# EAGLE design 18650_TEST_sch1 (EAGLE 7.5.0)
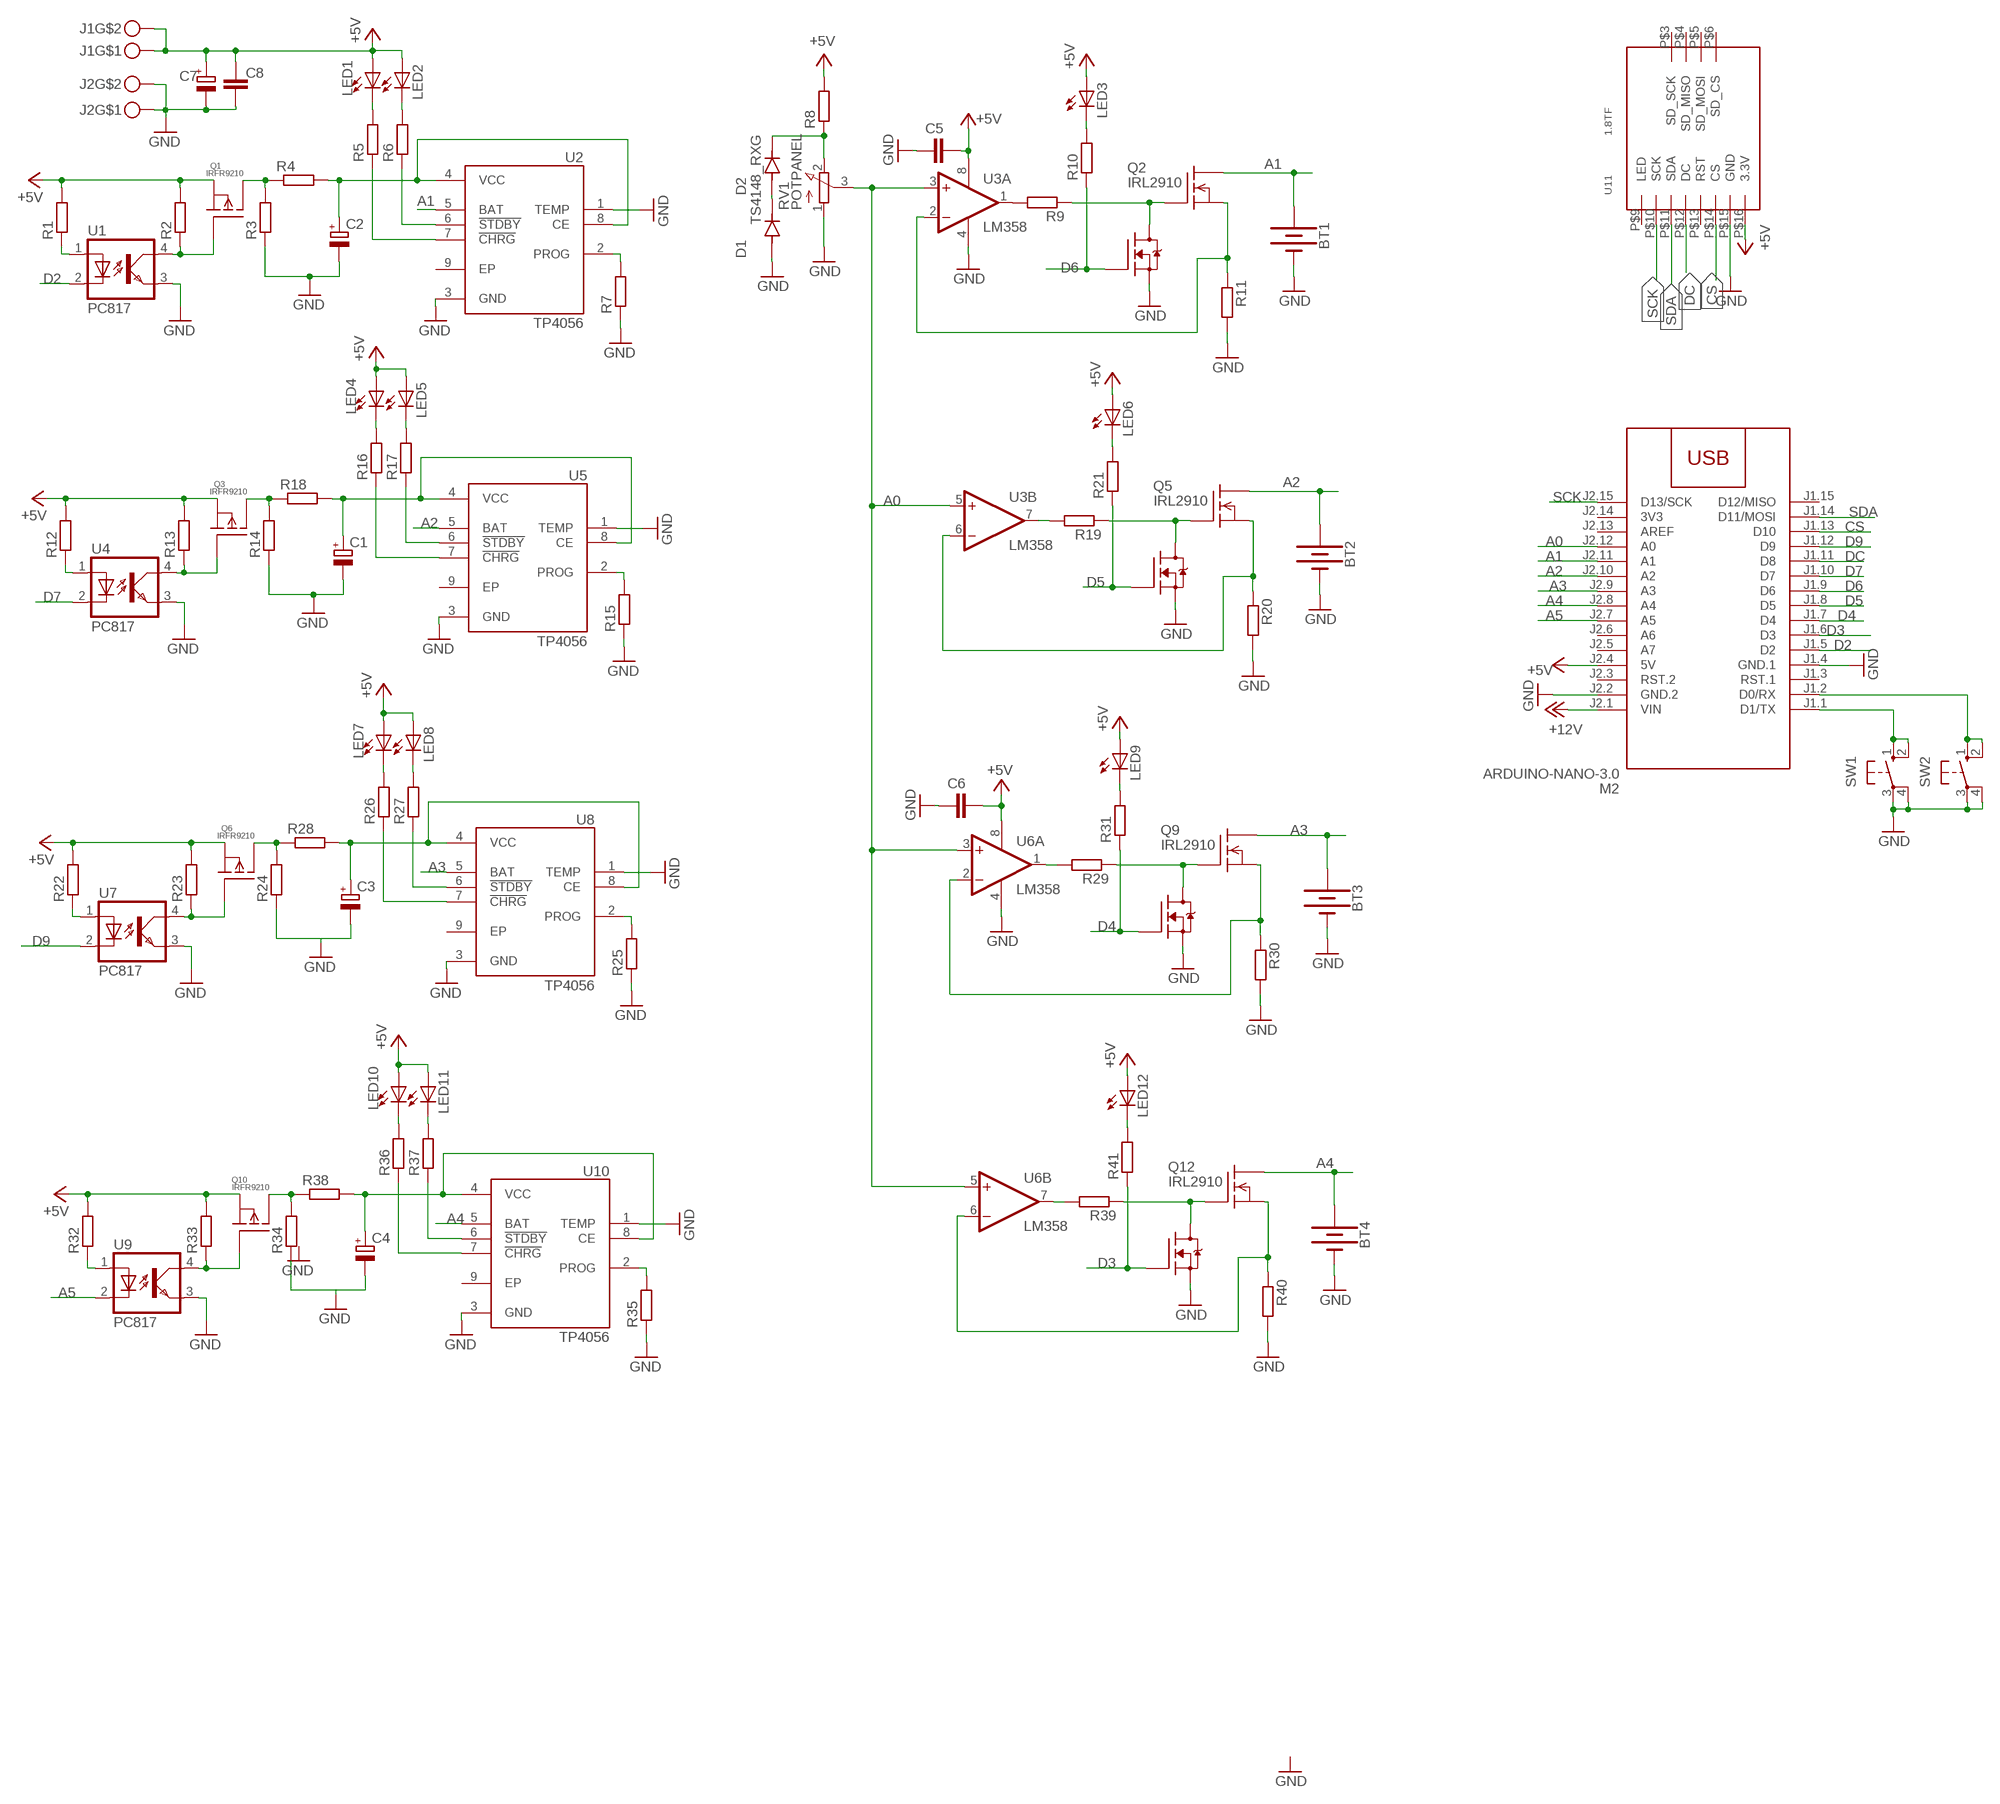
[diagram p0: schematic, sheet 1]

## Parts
BT1  BATTERY-18650  [BATTERY_18650-HOLDER]
BT2  BATTERY-18650  [BATTERY_18650-HOLDER]
BT3  BATTERY-18650  [BATTERY_18650-HOLDER]
BT4  BATTERY-18650  [BATTERY_18650-HOLDER]
C1  CPOL-EUSMCB  [SMC_B]
C2  CPOL-EUSMCB  [SMC_B]
C3  CPOL-EUSMCB  [SMC_B]
C4  CPOL-EUSMCB  [SMC_B]
C5  C-EUC1206  [C1206]
C6  C-EUC1206  [C1206]
C7  CPOL-EUSMCB  [SMC_B]
C8  C-EUC1206  [C1206]
D1  TS4148_RXG  [DIO_TS4148_RXG]
D2  TS4148_RXG  [DIO_TS4148_RXG]
J1  MKDSN1,5-2-5,08  [MKDSN1,5-2-5,08]
J2  MKDSN1,5-2-5,08  [MKDSN1,5-2-5,08]
LED1  LED5MM  [LED5MM]
LED2  LED5MM  [LED5MM]
LED3  LED5MM  [LED5MM]
LED4  LED5MM  [LED5MM]
LED5  LED5MM  [LED5MM]
LED6  LED5MM  [LED5MM]
LED7  LED5MM  [LED5MM]
LED8  LED5MM  [LED5MM]
LED9  LED5MM  [LED5MM]
LED10  LED5MM  [LED5MM]
LED11  LED5MM  [LED5MM]
LED12  LED5MM  [LED5MM]
M2  ARDUINO-NANO-3.0  [ARDUINO-NANO-3.0]
Q1  IRFR9210  [D2PACK]
Q2  IRL2910  SUP75N06-08  [TO220]
Q3  IRFR9210  [D2PACK]
Q4  ZVN3310F  [SOT23]
Q5  IRL2910  SUP75N06-08  [TO220]
Q6  IRFR9210  [D2PACK]
Q7  ZVN3310F  [SOT23]
Q8  ZVN3310F  [SOT23]
Q9  IRL2910  SUP75N06-08  [TO220]
Q10  IRFR9210  [D2PACK]
Q11  ZVN3310F  [SOT23]
Q12  IRL2910  SUP75N06-08  [TO220]
R1  R-EU_R1206  [R1206]
R2  R-EU_R1206  [R1206]
R3  R-EU_R1206  [R1206]
R4  R-EU_R2512  [R2512]
R5  R-EU_R1206  [R1206]
R6  R-EU_R1206  [R1206]
R7  R-EU_R1206  [R1206]
R8  R-EU_R1206  [R1206]
R9  R-EU_R1206  [R1206]
R10  R-EU_R1206  [R1206]
R11  R-EU_R2512  [R2512]
R12  R-EU_R1206  [R1206]
R13  R-EU_R1206  [R1206]
R14  R-EU_R1206  [R1206]
R15  R-EU_R1206  [R1206]
R16  R-EU_R1206  [R1206]
R17  R-EU_R1206  [R1206]
R18  R-EU_R2512  [R2512]
R19  R-EU_R1206  [R1206]
R20  R-EU_R2512  [R2512]
R21  R-EU_R1206  [R1206]
R22  R-EU_R1206  [R1206]
R23  R-EU_R1206  [R1206]
R24  R-EU_R1206  [R1206]
R25  R-EU_R1206  [R1206]
R26  R-EU_R1206  [R1206]
R27  R-EU_R1206  [R1206]
R28  R-EU_R2512  [R2512]
R29  R-EU_R1206  [R1206]
R30  R-EU_R2512  [R2512]
R31  R-EU_R1206  [R1206]
R32  R-EU_R1206  [R1206]
R33  R-EU_R1206  [R1206]
R34  R-EU_R1206  [R1206]
R35  R-EU_R1206  [R1206]
R36  R-EU_R1206  [R1206]
R37  R-EU_R1206  [R1206]
R38  R-EU_R2512  [R2512]
R39  R-EU_R1206  [R1206]
R40  R-EU_R2512  [R2512]
R41  R-EU_R1206  [R1206]
RV1  POTPANEL  [POTPANELP231]
SW1  40-XX  [B3F-40XX]
SW2  40-XX  [B3F-40XX]
U1  PC817  [DIL04]
U2  TP4056  [SOP127P600X175-9N]
U3  LM358  OPA2134PA  [DIL08]
U4  PC817  [DIL04]
U5  TP4056  [SOP127P600X175-9N]
U6  LM358  OPA2134PA  [DIL08]
U7  PC817  [DIL04]
U8  TP4056  [SOP127P600X175-9N]
U9  PC817  [DIL04]
U10  TP4056  [SOP127P600X175-9N]
U11  1.8TF  [1.8TFT]

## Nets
+5V: C5.1 C6.1 C7.+ C8.1 J1.1 J1.2 LED1.A LED2.A LED3.A LED4.A LED5.A LED6.A LED7.A LED8.A LED9.A LED10.A LED11.A LED12.A M2.J2.4(5V) Q1.3(S) Q3.3(S) Q6.3(S) Q10.3(S) R1.2 R2.2 R8.2 R12.2 R13.2 R22.2 R23.2 R32.2 R33.2 U3.8(A:V+) U6.8(A:V+) U11.P$16(3.3V)
+12V: M2.J2.1(VIN)
A0: M2.J2.12(A0) RV1.3(S) U3.3(A:+IN) U3.5(B:+IN) U6.3(A:+IN) U6.5(B:+IN)
A1: BT1.PWR@1(+) M2.J2.11(A1) Q2.2(D) U2.5(BAT)
A2: BT2.PWR@1(+) M2.J2.10(A2) Q5.2(D) U5.5(BAT)
A3: BT3.PWR@1(+) M2.J2.9(A3) Q9.2(D) U8.5(BAT)
A4: BT4.PWR@1(+) M2.J2.8(A4) Q12.2(D) U10.5(BAT)
A5: M2.J2.7(A5) U9.2(C)
CS: M2.J1.13(D10) U11.P$14(CS)
D2: M2.J1.5(D2) U1.2(C)
D3: M2.J1.6(D3) Q11.2(G) R41.1
D4: M2.J1.7(D4) Q8.2(G) R31.1
D5: M2.J1.8(D5) Q4.2(G) R21.1
D6: M2.J1.9(D6) Q7.2(G) R10.1
D7: M2.J1.10(D7) U4.2(C)
D9: M2.J1.12(D9) U7.2(C)
DC: M2.J1.11(D8) U11.P$12(DC)
GND: BT1.GND@1(-) BT2.GND@1(-) BT3.GND@1(-) BT4.GND@1(-) C1.- C2.- C3.- C4.- C5.2 C6.2 C7.- C8.2 D1.A J2.1 J2.2 M2.J1.4(GND.1) M2.J2.2(GND.2) Q4.3(S) Q7.3(S) Q8.3(S) Q11.3(S) R3.1 R7.1 R11.2 R14.1 R15.1 R20.2 R24.1 R25.1 R30.2 R34.1 R35.1 R40.2 RV1.1(A) SW1.3(P) SW1.4(P1) SW2.3(P) SW2.4(P1) U1.3(EMIT) U2.1(TEMP) U2.3(GND) U3.4(A:V-) U4.3(EMIT) U5.1(TEMP) U5.3(GND) U6.4(A:V-) U7.3(EMIT) U8.1(TEMP) U8.3(GND) U9.3(EMIT) U10.1(TEMP) U10.3(GND) U11.P$15(GND)
N$1: R7.2 U2.2(PROG)
N$2: LED1.K(C) R5.2
N$3: LED2.K(C) R6.2
N$4: R5.1 U2.7(!CHRG)
N$5: R6.1 U2.6(!STDBY)
N$6: Q1.2(D) R3.2 R4.1
N$7: M2.J1.1(D1/TX) SW1.1(S) SW1.2(S1)
N$8: M2.J1.2(D0/RX) SW2.1(S) SW2.2(S1)
N$9: R1.1 U1.1(A)
N$11: R12.1 U4.1(A)
N$12: Q1.1(G) R2.1 U1.4(COL)
N$13: C2.+ R4.2 U2.4(VCC) U2.8(CE)
N$14: Q3.1(G) R13.1 U4.4(COL)
N$15: C1.+ R18.2 U5.4(VCC) U5.8(CE)
N$16: R15.2 U5.2(PROG)
N$17: LED4.K(C) R16.2
N$18: LED5.K(C) R17.2
N$19: R16.1 U5.7(!CHRG)
N$20: R17.1 U5.6(!STDBY)
N$21: Q3.2(D) R14.2 R18.1
N$22: R19.2 U3.7(B:OUT)
N$23: Q4.1(D) Q5.1(G) R19.1
N$24: Q5.3(S) R20.1 U3.6(B:-IN)
N$25: LED6.K(C) R21.2
N$28: R22.1 U7.1(A)
N$29: Q6.1(G) R23.1 U7.4(COL)
N$30: C3.+ R28.2 U8.4(VCC) U8.8(CE)
N$31: R25.2 U8.2(PROG)
N$32: LED7.K(C) R26.2
N$33: LED8.K(C) R27.2
N$34: R26.1 U8.7(!CHRG)
N$35: R27.1 U8.6(!STDBY)
N$36: Q6.2(D) R24.2 R28.1
N$37: Q8.1(D) Q9.1(G) R29.1
N$38: Q9.3(S) R30.1 U6.2(A:-IN)
N$39: LED9.K(C) R31.2
N$40: R29.2 U6.1(A:OUT)
N$42: R32.1 U9.1(A)
N$43: Q10.1(G) R33.1 U9.4(COL)
N$44: C4.+ R38.2 U10.4(VCC) U10.8(CE)
N$45: R35.2 U10.2(PROG)
N$46: LED10.K(C) R36.2
N$47: LED11.K(C) R37.2
N$48: R36.1 U10.7(!CHRG)
N$49: R37.1 U10.6(!STDBY)
N$50: Q10.2(D) R34.2 R38.1
N$51: Q11.1(D) Q12.1(G) R39.1
N$52: Q12.3(S) R40.1 U6.6(B:-IN)
N$53: LED12.K(C) R41.2
N$55: R39.2 U6.7(B:OUT)
N$58: D2.C(K) R8.1 RV1.2(E)
N$59: D1.C(K) D2.A
N$60: R9.2 U3.1(A:OUT)
N$61: Q2.1(G) Q7.1(D) R9.1
N$62: Q2.3(S) R11.1 U3.2(A:-IN)
N$91: LED3.K(C) R10.2
SCK: M2.J2.15(D13/SCK) U11.P$10(SCK)
SDA: M2.J1.14(D11/MOSI) U11.P$11(SDA)
Unconnected: M2.J1.3(RST.1) M2.J1.15(D12/MISO) M2.J2.3(RST.2) M2.J2.5(A7) M2.J2.6(A6) M2.J2.13(AREF) U2.9(EP) U5.9(EP) U8.9(EP) U10.9(EP) U11.P$3(SD_SCK) U11.P$4(SD_MISO) U11.P$5(SD_MOSI) U11.P$6(SD_CS) U11.P$9(LED) U11.P$13(RST)

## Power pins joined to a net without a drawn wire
3V3: M2.J2.14(3V3)

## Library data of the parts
BT1-BT4 = SparkFun-Batteries:BATTERY: Battery - Single Cell; PROD_ID: BATT-12327; SF_SKU: PRT-13113
C1-C4 C7 = rcl:CPOL-EU: POLARIZED CAPACITOR, European symbol
C5 C6 C8 = rcl:C-EU: CAPACITOR, European symbol
D1 D2 = TS4148_RXG:TS4148_RXG: Check availability Check availability Check availability; AVAILABILITY: In Stock; CHECK_PRICES: https://www.snapeda.com/parts/TS4148%20RXG/Taiwan+Semiconductor/view-part/?ref=eda; DESCRIPTION: 1206 (Ceramics) 75V 0.15A Switching Diode & Array; MF: Taiwan Semiconductor; MP: TS4148 RXG; PACKAGE: 1206-2 Taiwan Semiconductor; PRICE: None; SNAPEDA_LINK: https://www.snapeda.com/parts/TS4148%20RXG/Taiwan+Semiconductor/view-part/?ref=snap
J1 J2 = con-phoenix-508:MKDSN1,5-2-5,08
LED1-LED12 = led:LED: LED
M2 = diy-modules:ARDUINO-NANO-3.0: Arduino Nano 3.0 and compatible devices More details available here: https://www.arduino.cc/en/Main/ArduinoBoardNano Click here to find device on ebay.com
Q1 Q3 Q6 Q10 = IRFR9210:IRFR9210: Check availability; AVAILABILITY: In Stock; CHECK_PRICES: https://www.snapeda.com/parts/IRFR9210/Vishay+Siliconix/view-part/?ref=eda; DESCRIPTION: P-Channel 200 V 1.9A (Tc) 2.5W (Ta), 25W (Tc) Surface Mount D-Pak; MF: Vishay; MP: IRFR9210; PACKAGE: TO-252-3 Infineon; PRICE: None; SNAPEDA_LINK: https://www.snapeda.com/parts/IRFR9210/Vishay+Siliconix/view-part/?ref=snap
Q2 Q5 Q9 Q12 = transistor-fet:SUP75N06-08: N-Channel Enhancement MOSFET 60V; 75A; 0,008Ohm
Q4 Q7 Q8 Q11 = transistor-fet:ZVN3310F
R1-R41 = rcl:R-EU_: RESISTOR, European symbol
RV1 = pot:POTPANEL
SW1 SW2 = switch-omron:40-XX: OMRON SWITCH; MF: OMRON COMPONENTS USA; MPN: B3F-4000; OC_FARNELL: 176434; OC_NEWARK: 36K3105
U1 U4 U7 U9 = optocoupler:PC817: SHARP OPTO COUPLER; MPN: PC817X4J000F; OC_FARNELL: 9707727; OC_NEWARK: 97K7059
U2 U5 U8 U10 = TP4056:TP4056: Check availability; AVAILABILITY: Not in stock; CHECK_PRICES: https://www.snapeda.com/parts/TP4056/NanJing+Top+Power+ASIC+Corp./view-part/?ref=eda; DESCRIPTION: Complete single cell Li-Ion battery with a constant current / constant voltage linear charger; MF: NanJing Top Power ASIC Corp.; MP: TP4056; PACKAGE: Package; PRICE: None; SNAPEDA_LINK: https://www.snapeda.com/parts/TP4056/NanJing+Top+Power+ASIC+Corp./view-part/?ref=snap
U3 U6 = linear:OPA2*: Dual Operational Amplifier Low Power, Single-Supply, Rail-To-Rail Operational Amplifier Source: http://focus.ti.com/lit/ds/symlink/opa2345.pdf http://focus.ti.com .. opa241.pdf http://focus.ti.com/lit/ds/symlink/opa2134.pdf
U11 = tft_1_8_1_44_oled_0_96:1.8TF

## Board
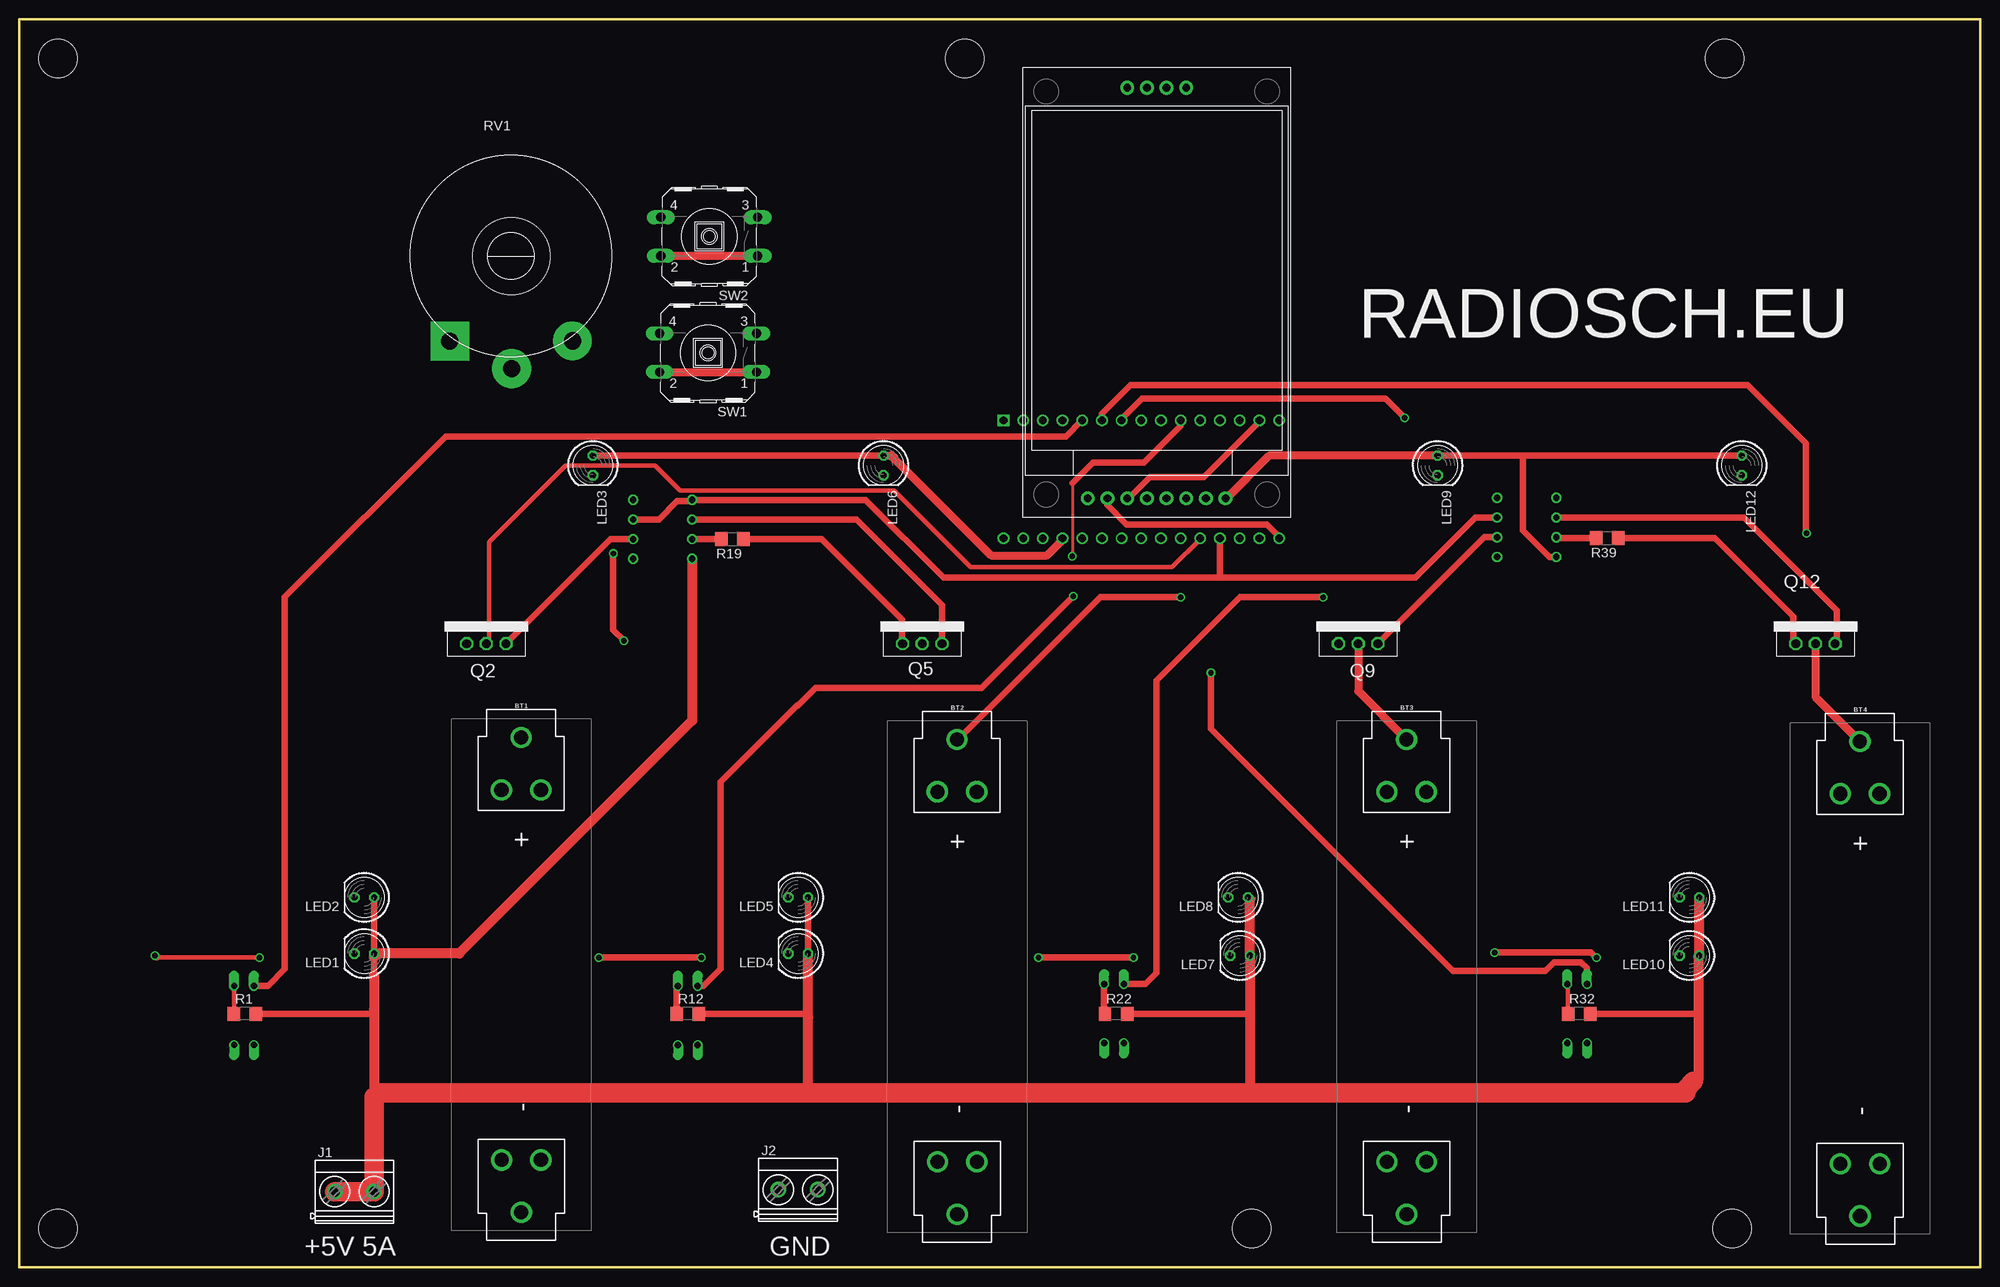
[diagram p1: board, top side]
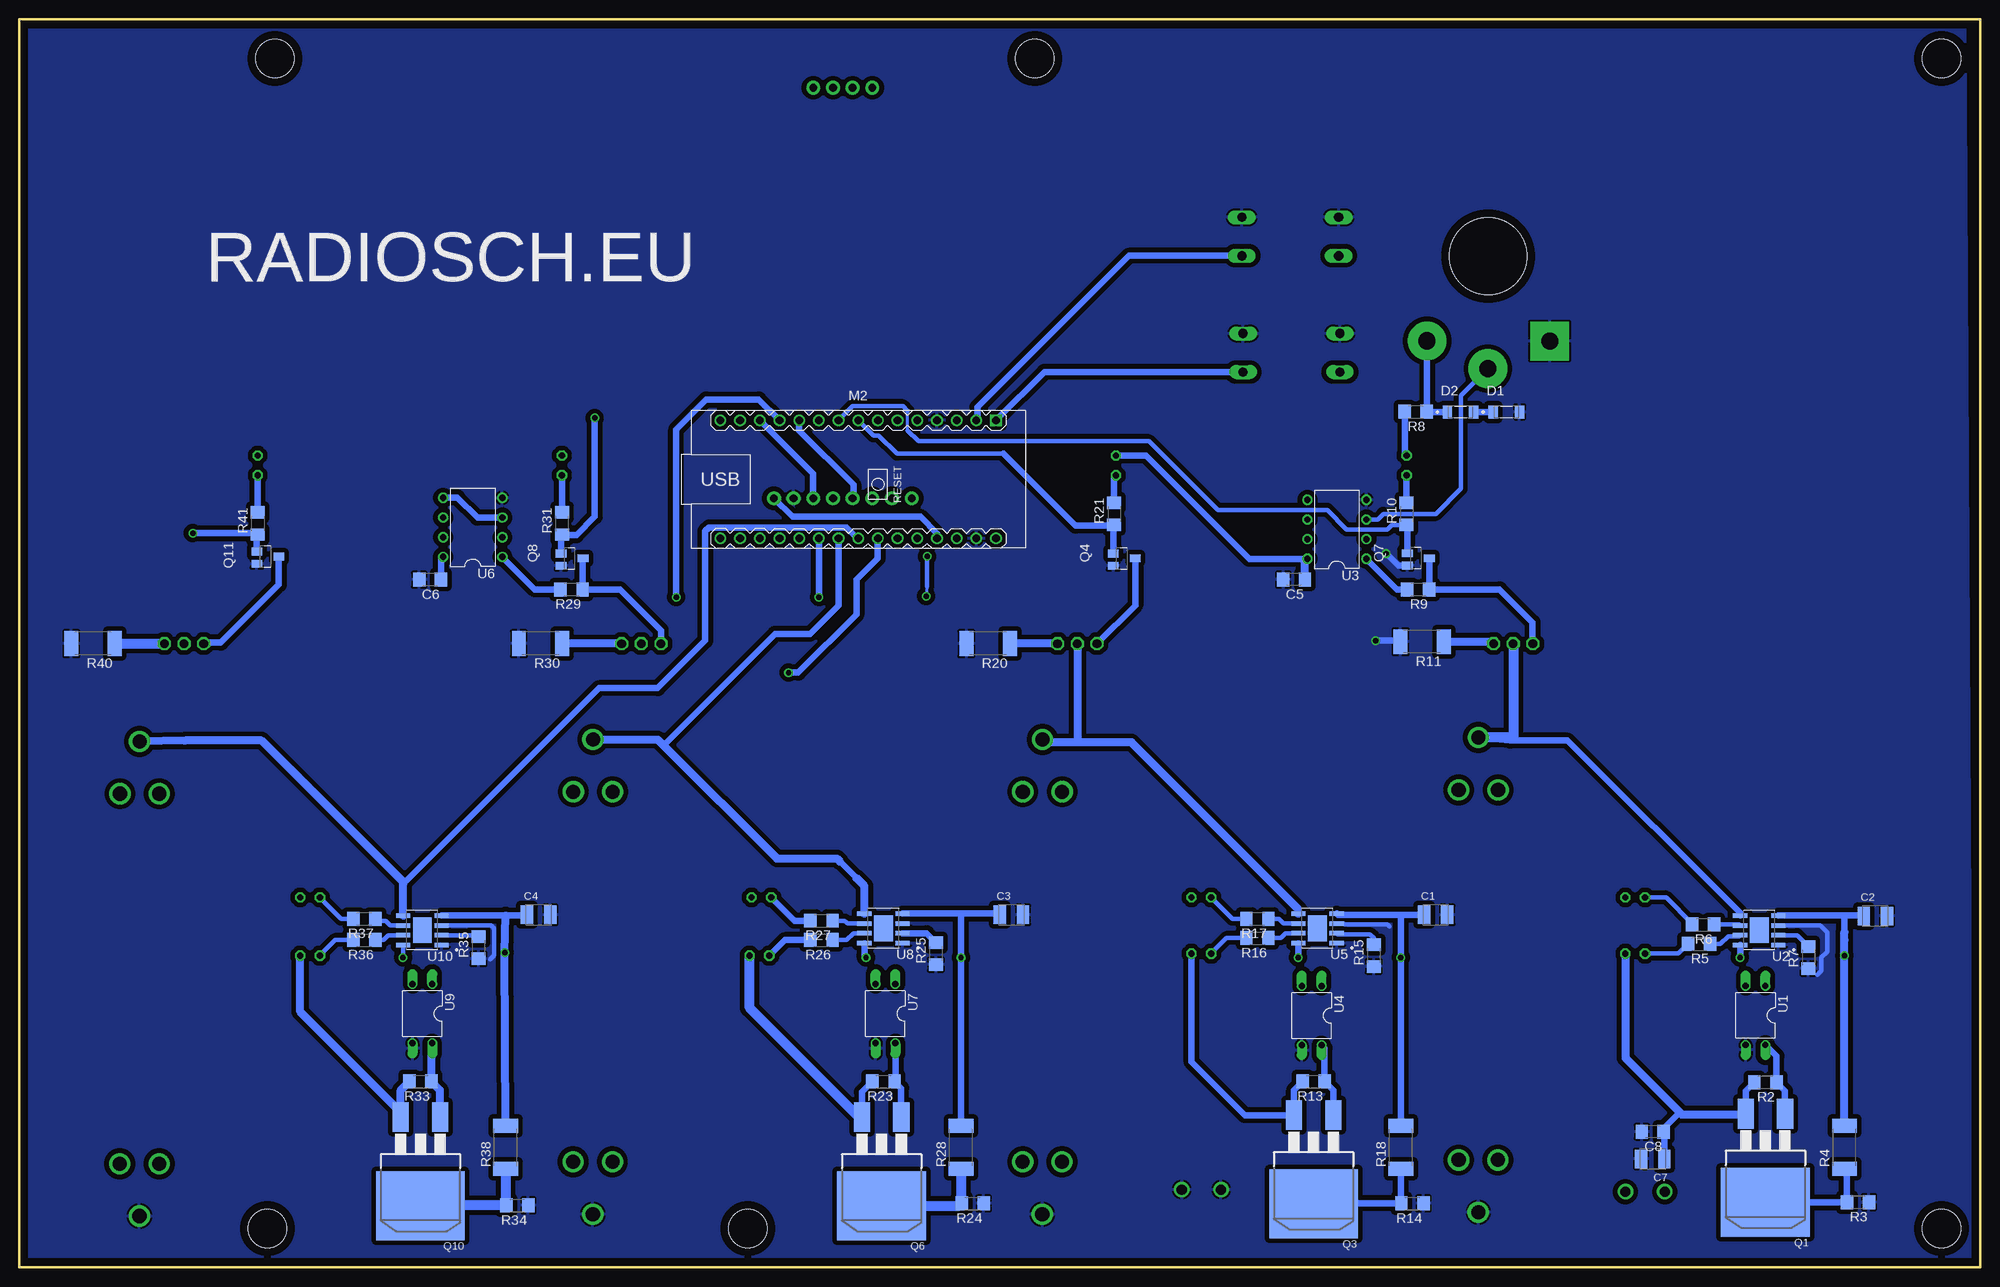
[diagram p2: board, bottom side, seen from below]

Size 253 x 161.06 mm. Coordinates in mm from the lower left corner, seen from the top.
Outline: 0,0 253,0 253,161.06 0,161.06 0,0
Copper layers (1*16): Top 0.035mm / dielectric 1.5mm / Bottom 0.035mm
Design rules "default": minimum track width 10mil, minimum drill 24mil, track to track 8mil, track to pad 8mil, pad to pad 8mil, via to via 8mil, smd to smd 8mil, copper to edge 40mil, drill to drill 8mil, minimum pad ring 10mil, minimum via ring 8mil, stop-mask expansion 4mil, vias tented up to drill 0mil, thermal gap 10mil
Holes 10 mm at 63.5,130.5
Holes 5 mm at 5,156 5,5 122,156 159,5 221,5 220,156

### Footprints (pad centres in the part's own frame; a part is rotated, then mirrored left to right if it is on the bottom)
BATTERY_18650-HOLDER = drill 1.829: GND@1 30.628,0.01; GND@2 23.88,2.55; GND@3 23.88,-2.53; PWR@1 -30.628,-0.01; PWR@2 -23.88,2.53; PWR@3 -23.88,-2.55
SMC_B = smd 1.6 x 2.4: + -1.5,0; - 1.5,0
C1206 = smd 1.6 x 1.8: 1 -1.4,0; 2 1.4,0
DIO_TS4148_RXG = smd 1.2 x 1.7: A 1.7,0; C -1.7,0
MKDSN1,5-2-5,08 = drill 1.3 pad 2: 1 -2.561,0.025; 2 2.519,0.025
LED5MM = drill 0.813 octagon: A -1.27,0; K 1.27,0
ARDUINO-NANO-3.0 = drill 1 square: J1.1 17.78,7.62 | drill 1: J1.2 15.24,7.62; J1.3 12.7,7.62; J1.4 10.16,7.62; J1.5 7.62,7.62; J1.6 5.08,7.62; J1.7 2.54,7.62; J1.8 0,7.62; J1.9 -2.54,7.62; J1.10 -5.08,7.62; J1.11 -7.62,7.62; J1.12 -10.16,7.62; J1.13 -12.7,7.62; J1.14 -15.24,7.62; J1.15 -17.78,7.62; J2.1 17.78,-7.62; J2.2 15.24,-7.62; J2.3 12.7,-7.62; J2.4 10.16,-7.62; J2.5 7.62,-7.62; J2.6 5.08,-7.62; J2.7 2.54,-7.62; J2.8 0,-7.62; J2.9 -2.54,-7.62; J2.10 -5.08,-7.62; J2.11 -7.62,-7.62; J2.12 -10.16,-7.62; J2.13 -12.7,-7.62; J2.14 -15.24,-7.62; J2.15 -17.78,-7.62
D2PACK = smd 2.083 x 3.81: 1 -2.54,-8.89; 3 2.54,-8.89 | smd 11.43 x 8.89: 2 0,2.54
TO220 = drill 1.118 octagon: 1 -2.54,0; 2 0,0; 3 2.54,0
SOT23 = smd 1 x 1.4: 1 0,1.735; 2 -0.632,-1.1; 3 0.95,-1.1
R1206 = smd 1.6 x 1.803: 1 -1.422,0; 2 1.422,0
R2512 = smd 1.8 x 3.2: 1 -2.8,0; 2 2.8,0
POTPANELP231 = drill 2.2 pad 5 square: 1 -7.85,-11 | drill 2.2 pad 5: 2 7.97,-10.96; 3 0.11,-14.54
B3F-40XX = drill 1.194 long: 1 -6.248,2.489; 2 6.248,2.489; 3 -6.248,-2.489; 4 6.248,-2.489
DIL04 = drill 0.813 offset: 1 -1.27,-3.81; 2 1.27,-3.81; 3 1.27,3.81; 4 -1.27,3.81
SOP127P600X175-9N = smd 1.97 x 0.6: 1 -2.475,1.905; 2 -2.475,0.635; 3 -2.475,-0.635; 4 -2.475,-1.905; 5 2.475,-1.905; 6 2.475,-0.635; 7 2.475,0.635; 8 2.475,1.905 | smd 2.413 x 3.302: 9 0,0
DIL08 = drill 0.813 pad 1.27: 1 -3.81,-3.81; 2 -1.27,-3.81; 3 1.27,-3.81; 4 3.81,-3.81; 5 3.81,3.81; 6 1.27,3.81; 7 -1.27,3.81; 8 -3.81,3.81
1.8TFT = drill 1 pad 1.778: P$3 55.5,21.05; P$4 55.5,18.52; P$5 55.5,15.98; P$6 55.5,13.44; P$9 2.5,26.14; P$10 2.5,23.6; P$11 2.5,21.06; P$12 2.5,18.52; P$13 2.5,15.98; P$14 2.5,13.44; P$15 2.5,10.9; P$16 2.5,8.36

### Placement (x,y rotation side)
BT1  64.75,37.75 270 top
BT2  121,37.5 270 top
BT3  179,37.5 270 top
BT4  237.5,37.25 270 top
C1  70.25,45.5 0 bottom
C2  13.51,45.35 0 bottom
C3  125,45.5 0 bottom
C4  186,45.5 0 bottom
C5  88.52,88.76 180 bottom
C6  200,88.75 180 bottom
C7  42.25,14 180 bottom
C8  42.25,17.5 180 bottom
D1  61.12,110.39 0 bottom
D2  67.05,110.39 0 bottom
J1  43.25,9.75 0 top
J2  100.5,10 0 top
LED1  44.5,40.5 180 top
LED2  44.5,47.75 180 top
LED3  74,103.5 270 top
LED4  100.5,40.5 180 top
LED5  100.5,47.75 180 top
LED6  111.5,103.5 270 top
LED7  157.5,40.25 180 top
LED8  157.25,47.75 180 top
LED9  183,103.5 270 top
LED10  215.5,40.25 180 top
LED11  215.5,47.75 180 top
LED12  222.25,103.5 270 top
M2  144.76,101.7 0 bottom
Q1  27.71,10.93 180 bottom
Q2  60.25,80.5 0 top
Q3  86,10.75 180 bottom
Q4  110.75,91.5 270 bottom
Q5  116.5,80.5 0 top
Q6  141.75,10.5 180 bottom
Q7  72.81,91.52 270 bottom
Q8  182,91.5 270 bottom
Q9  172.75,80.5 0 top
Q10  201.25,10.5 180 bottom
Q11  221.25,91.75 270 bottom
Q12  231.75,80.5 0 top
R1  29.11,32.73 0 top
R2  27.71,23.9 180 bottom
R3  15.76,8.43 180 bottom
R4  17.5,15.5 90 bottom
R5  36.25,41.75 180 bottom
R6  35.75,44.25 180 bottom
R7  22.16,40 90 bottom
R8  72.81,110.43 180 bottom
R9  72.5,87.5 180 bottom
R10  74,97.25 90 bottom
R11  72,80.75 180 bottom
R12  86.25,32.75 0 top
R13  86,24 180 bottom
R14  73.25,8.25 180 bottom
R15  78.25,40.25 90 bottom
R16  93.25,42.5 180 bottom
R17  93.25,45 180 bottom
R18  74.75,15.5 90 bottom
R19  92,94 180 top
R20  128,80.5 180 bottom
R21  111.75,97.25 90 bottom
R22  141.5,32.75 0 top
R23  141.5,24 180 bottom
R24  130,8.25 180 bottom
R25  134.75,40.5 90 bottom
R26  149.5,42.25 180 bottom
R27  149.5,44.75 180 bottom
R28  131.5,15.5 90 bottom
R29  181.75,87.5 180 bottom
R30  185.75,80.5 180 bottom
R31  183,96 90 bottom
R32  201.25,32.75 0 top
R33  201.25,24 180 bottom
R34  188.75,8 180 bottom
R35  193.75,41.25 90 bottom
R36  208.5,42.25 180 bottom
R37  208.5,45 180 bottom
R38  190.25,15.5 90 bottom
R39  204.88,94.12 180 top
R40  243.5,80.5 180 bottom
R41  222.25,96 90 bottom
RV1  63.4,130.53 0 top
SW1  88.86,118.03 180 top
SW2  89.02,133.03 180 top
U1  28.98,32.52 180 bottom
U2  28.5,43.5 180 bottom
U3  83,95.25 90 bottom
U4  86.25,32.5 180 bottom
U5  85.5,43.75 180 bottom
U6  194.5,95.5 90 bottom
U7  141.25,32.75 180 bottom
U8  141.5,43.75 180 bottom
U9  201,32.75 180 bottom
U10  201,43.5 180 bottom
U11  164,96.75 90 top

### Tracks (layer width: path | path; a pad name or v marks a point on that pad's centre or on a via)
+5V
  Top 0.813: 45.77,37.75 45.77,40 LED1.A LED2.A | LED5.A LED4.A 101.75,40.48 101.75,37 | R12.2 101.77,32.75 101.77,32.25 | R1.2 45.77,32.73 45.77,33.25 | R22.2 158.52,32.75 158.77,32.5 | R32.2 216.62,32.75 | LED3.A LED6.A | LED9.A 193.75,104.77 | 193.75,104.77 LED12.A | U6.8 197.44,91.69 194,95.12 194,104.52 193.75,104.77
  Top 1.016: LED6.A 112.48,104.77 125.38,91.88 132.62,91.88 134.6,93.85 M2.J2.4 | LED9.A 182.98,104.75 161.25,104.75 155.75,99.25 U11.P$16
  Top 1.27: 45.77,37.75 45.77,33.25 45.77,22 46.27,22.5 | 101.77,22.5 101.77,32.25 LED4.A | U3.8 86.81,70.56 56.75,40.5 46.27,40.5 45.77,40 | 159,22.5 158.77,22.73 158.77,32.5 LED7.A 158.77,47.5 LED8.A | LED11.A LED10.A 216.62,40.1 216.62,32.75 216.62,24.12 215,22.5 | J1.2
  Top 2.54: 46.27,22.5 101.77,22.5 159,22.5 214.5,22.5 215,23 | 45.77,22 J1.2 | J1.1 J1.2 | 215,23 216,24 | 215,22.5 215,23
  Bottom 0.813: Q1.3 30.25,22.78 R2.2 | R13.2 88.54,22.88 Q3.3 94.89,19.64 101.75,26.5 101.75,40.48 LED4.A | R23.2 144.29,22.63 Q6.3 | U3.8 94.3,91.44 107.62,104.77 LED6.A | C6.1 198.6,91.4 U6.8 | M2.J2.4 134.6,94.72 136.75,96.88 153.26,96.88 U11.P$16 | R8.2 74.24,105.01 LED3.A | C7.+ 40.75,17.4 C8.1 40.85,17.9 38.75,20
  Bottom 1.016: LED1.A 45.77,27.02 38.75,20 38.5,19.75 30.32,19.75 Q1.3 | C5.1 87.12,91.13 U3.8 | R33.2 203.79,22.88 Q10.3 203.79,20.04 216.75,33 216.75,40.23 LED10.A
  Bottom 1.27: Q6.3 144.66,19.39 158.77,33.5 LED7.A
A0
  Top 0.813: 79.17,96.5 U3.3 82.52,96.52 84.88,98.88 86.62,98.88 U3.5 109.19,99.06 119.25,89 155,89 | U6.3 190.67,96.75 187.88,96.75 180.12,89 155,89 | M2.J2.12 154.92,89.08 155,89
  Bottom 0.61: U3.3 77.73,96.52 77,97.25 70.25,97.25 67,100.5 67,112.5 RV1.3
  Bottom 0.813: U6.3 193.9,96.77 196.5,99.38 198.25,99.38 U6.5
A1
  Top 0.61: Q2.2 60.62,80.88 60.62,93.62 70.5,103.5 82,103.5 85.25,100.25 112.88,100.25 122.75,90.38 148.75,90.38 152.38,94 M2.J2.11
  Bottom 0.813: U2.5 30.98,45.73 53.25,68 60.62,68 BT1.PWR@1
  Bottom 1.27: Q2.2 60.25,68.37 BT1.PWR@1
A2  (via drill 0.7)
  Top 0.813: BT2.PWR@1 120.88,67.88 139.5,86.5 v149.84,86.5
  Bottom 0.813: v149.84,86.5 M2.J2.10
  Bottom 1.016: U5.5 87.97,46.23 109.5,67.75 116.25,67.75 | Q5.2 116.49,67.99 116.25,67.75 | 116.25,67.75 120.61,67.75 BT2.PWR@1
A3
  Top 1.016: Q9.2 172.75,74.37 BT3.PWR@1
  Bottom 0.813: 147.3,52.55 147.12,52.38 145,50.25 | M2.J2.9 147.3,85.45 151,81.75 155.5,81.75 169.88,67.38
  Bottom 1.016: U8.5 143.97,49.23 145,50.25 | BT3.PWR@1 170.63,68.13 169.88,67.38 155.25,52.75 147.5,52.75 147.12,52.38
A4
  Top 1.016: Q12.2 231.75,73.62 BT4.PWR@1
  Bottom 0.813: M2.J2.8 144.83,94.08 146.25,95.5 164,95.5 164.5,95 164.5,80.88 170.62,74.75 178.22,74.75 203.47,49.5
  Bottom 1.016: U10.5 203.47,49.5 203.47,49.73 221.75,68 231.61,68 BT4.PWR@1
A5  (via drill 0.7)
  Top 0.813: U9.2 202.25,36.58 202.25,38.62 201.5,39.38 198,39.38 196.88,38.25 185,38.25 153.75,69.5 v153.75,76.75
  Bottom 0.813: M2.J2.7 142.25,94.05 142.25,91.5 145,88.75 145,84.25 152.5,76.75 v153.75,76.75
CS
  Bottom 0.813: U11.P$14 150.56,102.42 M2.J1.13
D2
  Top 0.813: U1.2 32.08,36.33 34.25,38.5 34.25,86.5 55,107.25 135.07,107.25 M2.J1.5 137,109.46
D3  (via drill 0.7)
  Top 0.813: M2.J1.6 139.68,110.18 143.38,113.88 223,113.88 230.5,106.38 230.5,94.88 v230.62,94.75
  Bottom 0.813: Q11.2 222.35,94.48 R41.1 222.42,94.75 v230.62,94.75
D4  (via drill 0.7)
  Top 0.813: M2.J1.7 142.22,109.47 144.88,112.12 176.25,112.12 v178.75,109.62
  Bottom 0.813: Q8.2 183.1,94.48 R31.1 182.92,94.5 181.12,94.5 178.75,96.88 v178.75,109.62
D5
  Bottom 0.61: M2.J1.8 142.81,107.38 142.12,107.38 139.75,105 126,105
  Bottom 0.813: Q4.2 111.85,95.73 | 111.85,95.73 R21.1 | 111.85,95.73 116.73,95.73 126,105
D6
  Bottom 0.406: 138.38,108 138.38,110.5
  Bottom 0.61: R10.1 75.92,95.83 76.5,95.25 81.75,95.25 84.25,97.75 98.38,97.75 107.25,106.62 137,106.62 138.38,108 | 138.38,110.5 139,111.12 145.5,111.12 M2.J1.9
  Bottom 0.813: Q7.2 73.91,95.74 R10.1
D7  (via drill 0.7)
  Top 0.406: 135.88,101.25 v135.88,91.75
  Top 0.813: U4.2 88.31,36.31 90.5,38.5 90.5,62.62 100.38,72.5 100.5,72.5 102.75,74.75 124.12,74.75 v136,86.62 | M2.J1.10 149.84,108.59 145.12,103.88 138.5,103.88 135.88,101.25
  Bottom 0.406: 135.88,87.88 v136,86.62
  Bottom 0.61: v135.88,91.75 135.88,87.88
D9  (via drill 0.7)
  Top 0.813: U7.2 145.31,36.56 146.75,38 146.75,75.75 157.5,86.5 v168.25,86.5
  Bottom 0.813: v168.25,86.5 168.25,108.12 164.38,112 157.6,112 M2.J1.12
DC
  Bottom 0.813: M2.J1.11 152.38,108 145.38,101 145.38,99.36 U11.P$12
GND  (via drill 0.7)
  Top 0.813: v76.62,92.12 76.62,82.25 v78,80.88
  Bottom 0.61: U2.3 20.64,44.13 19.75,43.25 19.75,40.75 20.5,40 20.5,38.25 21,37.75 | U5.3 82.14,44.38 82,44.25 76.5,44.25 76.25,44 | U10.3 192.13,44.13 191.75,43.75 191.75,40.25 192.25,39.75
  Bottom 0.813: Q7.3 75.07,90.57 v76.62,92.12 | v78,80.88 74.92,80.88 R11.2
  pour Bottom (isolate 0.61): 2,174 292,173 291,-2 1,-1
N$1
  Bottom 0.61: U2.2 23.6,42.87 R7.2
N$2
  Bottom 0.61: LED1.K 38.92,40.5 R5.2
N$3
  Bottom 0.61: R6.2 37.17,44.42 40.5,47.75 LED2.K
N$4
  Bottom 0.61: R5.1 33.5,41.75 32.5,42.75 31.09,42.75 U2.7
N$5
  Bottom 0.61: R6.1 31.09,44.25 U2.6
N$6
  Bottom 0.813: Q1.2 17.22,8.39 R3.2 17.18,12.38 R4.1
N$7
  Top 1.016: SW1.2 SW1.1
  Bottom 0.813: SW1.1 120.75,115.55 M2.J1.1
N$8
  Top 1.016: SW2.2 SW2.1
  Bottom 0.813: SW2.1 109.83,130.55 129.38,111 129.38,109.47 M2.J1.2
N$9
  Top 0.61: R1.1 27.69,36.3 U1.1
N$11
  Top 0.813: R12.1 84.83,36.16 U4.1
N$12
  Bottom 0.813: Q1.1 25.18,22.78 R2.1 26.29,27.29 U1.4
N$13  (via drill 0.7)
  Top 0.61: v31,40 17.75,40
  Top 0.813: 17.75,40 v17.5,40.25
  Bottom 0.813: U2.4 17.75,45.41 | 17.75,45.41 15.06,45.41 C2.+ | 17.5,43.25 17.5,45.16 17.75,45.41 | U2.8 30.98,40.02 v31,40
  Bottom 1.016: R4.2 v17.5,40.25 17.5,42.25 17.5,43.25
N$14
  Bottom 0.813: Q3.1 83.46,22.88 R13.1 84.58,28.29 U4.4
N$15  (via drill 0.7)
  Top 0.813: v88,40 v74.75,40
  Bottom 0.813: U5.8 87.97,40.02 v88,40 | 74.75,45.5 v74.75,40 R18.2 | 74.75,45.5 82.87,45.5 U5.4 | C1.+ 74.75,45.5
N$16
  Bottom 0.61: R15.2 78.25,42.5 78.75,43 82.91,43 U5.2
N$17
  Bottom 0.61: R16.2 97.23,42.5 LED4.K
N$18
  Bottom 0.61: R17.2 96.48,45 LED5.K
N$19
  Bottom 0.61: U5.7 89.64,43.12 90.25,42.5 R16.1
N$20
  Bottom 0.61: U5.6 89.89,44.38 90.5,45 R17.1
N$21
  Bottom 0.813: Q3.2 86,8.25 R14.2 74.75,8.25 R18.1
N$22
  Top 0.813: R19.2 86.83,94 U3.7
N$23
  Top 0.813: R19.1 103.5,94 113.88,83.62 113.88,80.58 Q5.1
  Bottom 0.813: Q4.1 109.02,85.44 Q5.1
N$24
  Top 0.813: Q5.3 119.04,85.46 108,96.5 86.83,96.5 U3.6
  Bottom 1.016: Q5.3 R20.1
N$25
  Bottom 0.813: R21.2 111.75,101.98 LED6.K
N$28
  Top 0.813: U7.1 139.98,32.85 R22.1
N$29
  Bottom 0.813: U7.4 139.98,24.1 R23.1 139.21,23.13 Q6.1
N$30  (via drill 0.7)
  Top 0.813: v143.75,40 v131.5,40
  Bottom 0.813: U8.4 131.75,45.66 | 131.75,45.66 126.66,45.66 C3.+ | R28.2 v131.5,40 131.5,45.41 131.75,45.66 | U8.8 143.97,40.23 v143.75,40
N$31
  Bottom 0.813: U8.2 135.94,43.12 R25.2
N$32
  Bottom 0.813: R26.2 154.23,42.25 LED7.K
N$33
  Bottom 0.813: R27.2 152.98,44.75 LED8.K
N$34
  Bottom 0.61: U8.7 145.38,43.12 146.25,42.25 R26.1
N$35
  Bottom 0.61: U8.6 146.13,44.38 146.5,44.75 R27.1
N$36
  Bottom 1.27: Q6.2 131.71,7.96 R24.2 131.5,8.33 R28.1
N$37
  Bottom 0.813: Q9.1 170.21,82.21 175.5,87.5 R29.1 180.33,91.44 Q8.1
N$38
  Top 0.813: U6.2 189.02,94.23 Q9.3
  Bottom 1.016: Q9.3 R30.1
N$39
  Bottom 0.813: R31.2 LED9.K
N$40
  Bottom 0.813: R29.2 186.5,87.5 U6.1
N$42
  Top 0.61: R32.1 199.83,36.46 U9.1
N$43
  Bottom 1.016: Q10.1 198.71,22.88 R33.1 199.83,28.84 U9.4
N$44  (via drill 0.7)
  Top 0.813: v203.5,40 203.38,40 202.75,40.62 v190.38,40.62
  Bottom 0.61: U10.8 203.47,40.02 v203.5,40
  Bottom 0.813: U10.4 190.25,45.41 187.59,45.41 C4.+
  Bottom 1.016: R38.2 v190.38,40.62 190.25,45.41
N$45
  Bottom 0.61: U10.2 193.94,42.87 R35.2
N$46
  Bottom 0.61: R36.2 212.23,42.25 LED10.K
N$47
  Bottom 0.61: R37.2 211.48,45 LED11.K
N$48
  Bottom 0.61: U10.7 205.38,42.87 206,42.25 R36.1
N$49
  Bottom 0.61: U10.6 205.13,44.13 205.75,44.75 206.83,44.75 R37.1
N$50
  Bottom 1.27: Q10.2 201.21,8 R34.2 190.25,8.08 R38.1
N$51
  Top 0.813: R39.1 218.75,94.12 228.88,84 228.88,80.83 Q12.1
  Bottom 0.813: Q11.1 219.51,88.11 227,80.62 229.09,80.62 Q12.1
N$52
  Top 0.813: U6.6 222.48,96.77 234.5,84.75 234.5,80.71 Q12.3
  Bottom 1.27: R40.1 Q12.3
N$53
  Bottom 0.813: R41.2 LED12.K
N$55
  Top 0.813: R39.2 198.41,94.12 U6.7
N$58
  Bottom 0.813: D2.C 71.36,110.39 R8.1 71.36,110.46 RV1.2
N$59
  Bottom 0.813: D2.A D1.C
N$60
  Bottom 0.813: R9.2 75.25,87.5 U3.1
N$61
  Bottom 0.813: Q7.1 R9.1 | R9.1 | R9.1 62,87.5 57.75,83.25 57.75,80.54 Q2.1
N$62
  Top 0.813: U3.2 76.27,93.98 Q2.3
  Bottom 1.016: R11.1 63.04,80.75 Q2.3
N$91
  Bottom 0.813: R10.2 LED3.K
SCK
  Top 0.813: M2.J2.15 162.54,94.33 161,95.88 142.88,95.88 140.38,98.38 140.38,99.22 U11.P$10
SDA
  Top 0.813: U11.P$11 143.12,99.25 145.88,102 152.88,102 159.88,109 159.88,109.19 M2.J1.14

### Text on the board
tPlace: RADIOSCH.EU | +5V 5A | GND
bPlace: RADIOSCH.EU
